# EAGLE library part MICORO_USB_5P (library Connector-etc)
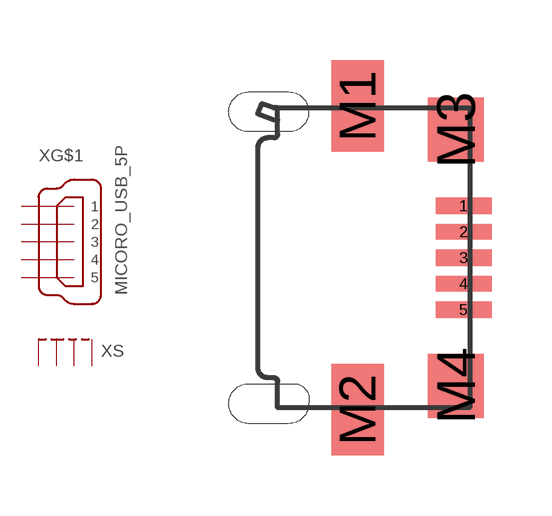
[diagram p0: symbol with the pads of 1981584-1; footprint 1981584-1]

Designator prefix X; gates G$1=MICRO-USB-5 S=SHIELD_4

## MICORO_USB_5P1981584-1  [1981584-1]
1  G$1:1  pas
2  G$1:2  pas
3  G$1:3  pas
4  G$1:4  pas
5  G$1:5  pas
M1  S:S1  pas
M2  S:S2  pas
M3  S:S3  pas
M4  S:S4  pas

## Footprint 1981584-1 (pad centres in mm)
smd 1.4 x 0.4: 1 2.65,1.3; 2 2.65,0.65; 3 2.65,0; 4 2.65,-0.65; 5 2.65,-1.3
smd 1.3 x 2.3: M1 0,3.8; M2 0,-3.8
smd 1.4 x 1.6: M3 2.45,3.2; M4 2.45,-3.2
